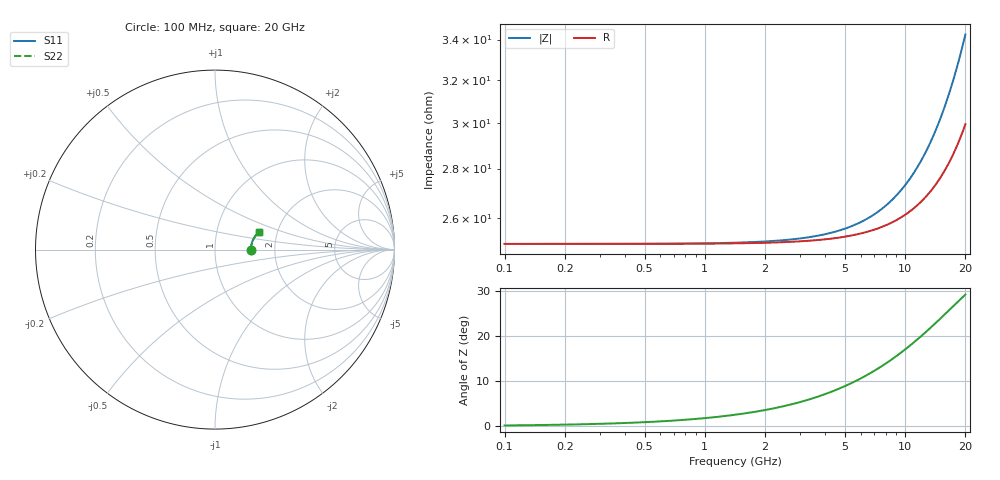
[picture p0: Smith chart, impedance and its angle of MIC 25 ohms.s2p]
! Vishay ElectroFilms Inc.
! MIC001 2500B - 25 Ohm in Series Configuration
! March 2012
# GHz S MA R 50
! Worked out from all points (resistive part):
!   233 points, 100 MHz to 20 GHz, reference 50 ohm
!   read as one part in series: R = 25 ohm at 102.3 MHz
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0.1  0.2 0.1  0.8 -0.0  0.8 -0.0  0.2 0.1
0.2436751  0.2 0.4  0.8 -0.1  0.8 -0.1  0.2 0.4
0.5937753  0.2001 0.9  0.8 -0.2  0.8 -0.2  0.2001 0.9
0.9375335  0.2001 1.3  0.7999 -0.3  0.7999 -0.3  0.2001 1.3
1.414214  0.2003 2.0  0.7998 -0.5  0.7998 -0.5  0.2003 2.0
2.284535  0.2009 3.3  0.7996 -0.8  0.7996 -0.8  0.2009 3.3
2.805834  0.2013 4.0  0.7993 -1.0  0.7993 -1.0  0.2013 4.0
3.446086  0.2019 4.9  0.799 -1.2  0.799 -1.2  0.2019 4.9
4.532574  0.2034 6.4  0.7982 -1.6  0.7982 -1.6  0.2034 6.4
5.695439  0.2053 8.0  0.7972 -2.1  0.7972 -2.1  0.2053 8.0
6.995058  0.208 9.7  0.7958 -2.5  0.7958 -2.5  0.208 9.7
7.664154  0.2095 10.6  0.7949 -2.8  0.7949 -2.8  0.2095 10.6
8.397251  0.2114 11.5  0.7939 -3.0  0.7939 -3.0  0.2114 11.5
9.630449  0.215 12.9  0.792 -3.5  0.792 -3.5  0.215 12.9
10.79537  0.2187 14.2  0.7899 -3.9  0.7899 -3.9  0.2187 14.2
12.10121  0.2234 15.6  0.7872 -4.4  0.7872 -4.4  0.2234 15.6
13.56501  0.2292 17.1  0.7838 -4.9  0.7838 -4.9  0.2292 17.1
14.52696  0.2333 17.9  0.7813 -5.3  0.7813 -5.3  0.2333 17.9
15.20587  0.2364 18.5  0.7795 -5.5  0.7795 -5.5  0.2364 18.5
16.66035  0.2434 19.7  0.7751 -6.1  0.7751 -6.1  0.2434 19.7
18.25396  0.2517 20.8  0.7699 -6.7  0.7699 -6.7  0.2517 20.8
20  0.2615 21.8  0.7634 -7.3  0.7634 -7.3  0.2615 21.8
